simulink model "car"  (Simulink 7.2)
settings: Solver=ode15s  StartTime=0.0  StopTime=60  RelTol=1e-3
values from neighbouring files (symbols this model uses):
  A_a = 1.5    [modelparam.m]
  b_f = 0.1    [modelparam.m]
  b_t = 0.1    [modelparam.m]
  brake_gain = 1.0e3    (= 1000)    [modelparam.m]
  Bx = Kxk/(Cx*Dx)    (= 12.5)    [modelparam.m]
  c_c = 30    [modelparam.m]
  c_d = 1    [modelparam.m]
  c_p = 15    [modelparam.m]
  c_r = 0.015    [modelparam.m]
  c_w = 0.30    (= 0.3)    [modelparam.m]
  Cx = 1.2    [modelparam.m]
  Dx = muX*Fz    (= 5886)    [modelparam.m]
  Ex = 0.8    [modelparam.m]
  g = 9.81    [modelparam.m]
  gearInertia = [0.13 0.09 0.07 0.05 0.04]    [modelparam.m]
  gearNumber = [1 2 3 4 5]    [modelparam.m]
  gearRatio = [3.4 2.2 1.5 1.1 0.9]    [modelparam.m]
  i_f = 3.4    [modelparam.m]
  init_d = init_v/r_w/3.6    (= 27.7777777778)    [modelparam.m]
  init_e = init_t*gearRatio(2)    [modelparam.m]
  init_f = init_d    (= 27.7777777778)    [modelparam.m]
  init_t = init_f*i_f    (= 94.4444444444)    [modelparam.m]
  init_T = 0    [modelparam.m]
  J_e = 0.2    [modelparam.m]
  J_f = 0.1    [modelparam.m]
  J_w = 0.6    [modelparam.m]
  k_c = 10e3    (= 10000)    [modelparam.m]
  k_d = 1e3    (= 1000)    [modelparam.m]
  k_p = 0.5e4    (= 5000)    [modelparam.m]
  mass = 1.5e3    (= 1500)    [modelparam.m]
  N_max = 7e3*pi/30    (= 733.038285838)    [modelparam.m]
  position = [0 1e6]    [modelparam.m]
  r_w = 0.30    (= 0.3)    [modelparam.m]
  Rho_a = 1.29    [modelparam.m]
  slope = [0 0]    [modelparam.m]
  T_max = 400    [modelparam.m]
  tau_d = 1e-3    (= 0.001)    [modelparam.m]
  tau_e = 0.1    [modelparam.m]
libraries: simulink x4

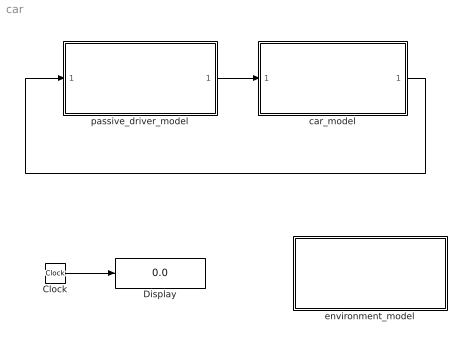
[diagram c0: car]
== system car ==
  Clock : Clock
  Display : Display
  car_model : Subsystem
  environment_model : Subsystem  AncestorBlock=capsim_lib/Environment/environment_model_jofr1  mask{Tamb=0, Pamb=0, pos=position, slope=slope}
      mask prompts: Tamb "Ambient Temperature [K]"; Pamb "Ambient Pressure [Pa]"; pos "positionvector in slope map [m]"; slope "slopevector in slope map [rad]"
      mask help: Environment settings
  passive_driver_model : Subsystem  AncestorBlock=capsim_lib/Driver/driver_model_template
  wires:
  car_model/1(vehicle fb out) -> passive_driver_model/1(vehicle fb in)
  passive_driver_model/1(driver cmd out) -> car_model/1(driver cmd in)
  Clock/1 -> Display/1

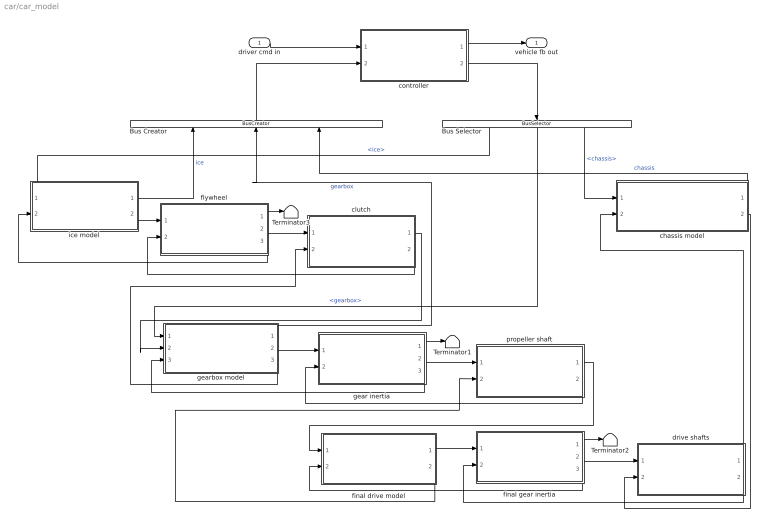
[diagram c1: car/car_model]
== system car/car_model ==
  driver cmd in : Inport  OutDataType=sfix(16)  OutScaling=2^0
  Bus Creator : BusCreator  Orientation=up  Inputs=3
  Bus Selector : BusSelector  Orientation=down  OutputSignals=ice,gearbox,chassis
  Terminator1 : Terminator
  Terminator2 : Terminator
  Terminator3 : Terminator
  chassis model : Subsystem  AncestorBlock=capsim_lib/Chassis/chassis_model_template
  clutch : Subsystem  AncestorBlock=capsim_lib/MechConverter/mechconverter_simple1_std  mask{mass=0, inertia=0, k_c=k_c, c_c=c_c}
      mask prompts: mass "Component mass [kg]"; inertia "Inertia [kg*m2]"; k_c "stiffness [Nm/rad]"; c_c "damping [Nms/rad]"
      mask help: Inertia
  controller : Subsystem  AncestorBlock=capsim_lib/Controller/controller_template
  drive shafts : Subsystem  AncestorBlock=capsim_lib/MechConverter/mechconverter_simple1_std  mask{mass=0, inertia=0, k_d=k_d, c_d=c_d}
      mask prompts: mass "Component mass [kg]"; inertia "Inertia [kg*m2]"; k_d "stiffness [Nm/rad]"; c_d "damping [Nms/rad]"
      mask help: Inertia
  final drive model : Subsystem  AncestorBlock=capsim_lib/Gearbox/gearbox_template
  final gear inertia : Subsystem  AncestorBlock=capsim_lib/Inertia/inertia_simple1_std  mask{mass=0, inertia=0, speedinit=init_f, angleinit=0}
      mask prompts: mass "Component mass [kg]"; inertia "Inertia [kg*m2]"; speedinit "Initial speed [rad/s]"; angleinit "Initial angle [rad]"
      mask help: Inertia
  flywheel : Subsystem  AncestorBlock=capsim_lib/Inertia/inertia_simple1_std  mask{mass=0, inertia=0, speedinit=init_e, angleinit=0}
      mask prompts: mass "Component mass [kg]"; inertia "Inertia [kg*m2]"; speedinit "Initial speed [rad/s]"; angleinit "Initial angle [rad]"
      mask help: Inertia
  gear inertia : Subsystem  AncestorBlock=capsim_lib/Inertia/inertia_simple1_std  mask{mass=0, inertia=0, speedinit=init_t, angleinit=0}
      mask prompts: mass "Component mass [kg]"; inertia "Inertia [kg*m2]"; speedinit "Initial speed [rad/s]"; angleinit "Initial angle [rad]"
      mask help: Inertia
  gearbox model : Subsystem  AncestorBlock=capsim_lib/Gearbox/gearbox_template
  ice model : Subsystem  AncestorBlock=capsim_lib/ICE/ice_model_template
  propeller shaft : Subsystem  AncestorBlock=capsim_lib/MechConverter/mechconverter_simple1_std  mask{mass=0, inertia=0, k_p=k_p, c_p=c_p}
      mask prompts: mass "Component mass [kg]"; inertia "Inertia [kg*m2]"; k_p "stiffness [Nm/rad]"; c_p "damping [Nms/rad]"
      mask help: Inertia
  vehicle fb out : Outport  OutDataType=sfix(16)  OutScaling=2^0
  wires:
  controller/1(vehicle fb out) -> vehicle fb out/1
  driver cmd in/1 -> controller/1(driver cmd in)
  controller/2(cmd out) -> Bus Selector/1
  Bus Creator/1 -> controller/2(sensor in)
  Bus Selector/1 -> ice model/1(cmd in)  "<ice>"
  Bus Selector/3 -> chassis model/1(cmd in)  "<chassis>"
  chassis model/1(sensor out) -> Bus Creator/3  "chassis"
  ice model/2(mech power out [Nm]) -> flywheel/1(mech in [Nm])
  flywheel/3(mech fb out [rad/s]) -> ice model/2(mech fb in [rad/s])
  flywheel/2(mech out [rad/s]) -> clutch/1(mech in [rad/s])
  clutch/2(mech fb out [Nm]) -> flywheel/2(mech fb in [Nm])
  clutch/1(mech out [Nm]) -> gearbox model/2(mech power in [Nm])
  gearbox model/2(mech power out [Nm]) -> gear inertia/1(mech in [Nm])
  gearbox model/3(mech fb out [rad/s]) -> clutch/2(mech fb in [rad/s])
  gear inertia/3(mech fb out [rad/s]) -> gearbox model/3(mech fb in [rad/s])
  gear inertia/2(mech out [rad/s]) -> propeller shaft/1(mech in [rad/s])
  propeller shaft/2(mech fb out [Nm]) -> gear inertia/2(mech fb in [Nm])
  propeller shaft/1(mech out [Nm]) -> final drive model/1(mech power in [Nm])
  final drive model/2(mech fb out [rad/s]) -> propeller shaft/2(mech fb in [rad/s])
  final drive model/1(mech power out [Nm]) -> final gear inertia/1(mech in [Nm])
  final gear inertia/2(mech out [rad/s]) -> drive shafts/1(mech in [rad/s])
  final gear inertia/3(mech fb out [rad/s]) -> final drive model/2(mech fb in [rad/s])
  drive shafts/1(mech out [Nm]) -> chassis model/2(mech power in [Nm])
  drive shafts/2(mech fb out [Nm]) -> final gear inertia/2(mech fb in [Nm])
  chassis model/2(mech fb out [rad/s]) -> drive shafts/2(mech fb in [rad/s])
  ice model/1(sensor out) -> Bus Creator/1  "ice"
  flywheel/1(sensor out) -> Terminator3/1
  gearbox model/1(sensor out) -> Bus Creator/2  "gearbox"
  gear inertia/1(sensor out) -> Terminator1/1
  final gear inertia/1(sensor out) -> Terminator2/1
  Bus Selector/2 -> gearbox model/1(cmd in)  "<gearbox>"

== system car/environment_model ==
  Compare To Constant : simulink/Logic and Bit Operations/Compare To Constant  SystemSampleTime=-1  relop=<  const=1  LogicOutDataTypeMode=uint8  ZeroCross=off
  Compare To Constant1 : simulink/Logic and Bit Operations/Compare To Constant  SystemSampleTime=-1  relop=<  const=1  LogicOutDataTypeMode=uint8  ZeroCross=off
  Constant2 : Constant  Value=pos(end)  OutDataType=sfix(16)  OutScaling=2^0
  Integrator : Integrator
  Logical Operator : Logic  Operator=OR  Inputs=3  AllPortsSameDT=off  OutDataTypeMode=boolean  OutDataTypeStr=boolean
  Relational Operator : RelationalOperator
  Stop Simulation1 : Stop
  To Workspace2 : ToWorkspace  VariableName=environmentout  SampleTime=-1  SaveFormat=Array
  slope as function of the distance : Lookup  InputValues=pos  Table=slope  LookUpMeth=Interpolation-Use End Values  OutDataType=sfix(16)  OutScaling=2^0
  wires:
  [speed] -> Integrator/1, Compare To Constant/1
  Integrator/1 -> slope as function of the distance/1, Relational Operator/1  "distance"
  slope as function of the distance/1 -> [slope], To Workspace2/1
  Constant2/1 -> Relational Operator/2
  Logical Operator/1 -> Stop Simulation1/1
  Relational Operator/1 -> Logical Operator/1
  Compare To Constant/1 -> Logical Operator/2
  [wheelspeed] -> Compare To Constant1/1
  Compare To Constant1/1 -> Logical Operator/3

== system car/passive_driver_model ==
  vehicle fb in : Inport  OutDataType=sfix(16)  OutScaling=2^0
  Bus Creator : BusCreator  Inputs=1
  Bus Selector : BusSelector  OutputSignals=velocity [m/s]
  From Workspace2 : FromWorkspace  VariableName=[InputT InputU]  SampleTime=0
  Terminator : Terminator
  driver cmd out : Outport  OutDataType=sfix(16)  OutScaling=2^0
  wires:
  vehicle fb in/1 -> Bus Selector/1
  Bus Creator/1 -> driver cmd out/1
  Bus Selector/1 -> Terminator/1  "<velocity [m/s]>"
  From Workspace2/1 -> Bus Creator/1  "Torque demand [%]"

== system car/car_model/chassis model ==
  cmd in : Inport  OutDataType=sfix(16)  OutScaling=2^0
  mech power in [Nm] : Inport  Port=2  OutDataType=sfix(16)  OutScaling=2^0
  chassis : Subsystem  mask{g=g, mass=mass, J_w=J_w, r_w=r_w, init_d=init_d, c_w=c_w, A_a=A_a, Rho_a=Rho_a, c_r=c_r, Bx=Bx, Cx=Cx, Dx=Dx, Ex=Ex}
      mask prompts: g "gravity constant [m/s^2]"; mass "vehicle mass [kg]"; J_w "wheel inertia [kg m^2]"; r_w "wheel radius [m]"; init_d "initial drive shaft speed [rad/s]"; c_w "air drag coefficient [-]"; A_a "max. vehicle cross section area [m^2]"; Rho_a "Air density [kg/m^3]"; c_r "rolling resistance coefficient [-]"; Bx "Magic Bx"; Cx "Magic Cx"; Dx "Magic Dx"; Ex "Magic Ex"
  local controller : Subsystem  mask{brake_gain=brake_gain}
      mask prompts: brake_gain "brake gain [Nm]"
  sensor out : Outport  OutDataType=sfix(16)  OutScaling=2^0
  mech fb out [rad/s] : Outport  Port=2  OutDataType=sfix(16)  OutScaling=2^0
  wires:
  local controller/2(ctrl out) -> chassis/1(ctrl in)
  cmd in/1 -> local controller/1(cmd in)
  local controller/1(sensor out) -> sensor out/1
  chassis/1(sensor out) -> local controller/2(sensor in)
  mech power in [Nm]/1 -> chassis/2(mech power in [Nm])
  chassis/2(mech fb out [rad/s]) -> mech fb out [rad/s]/1

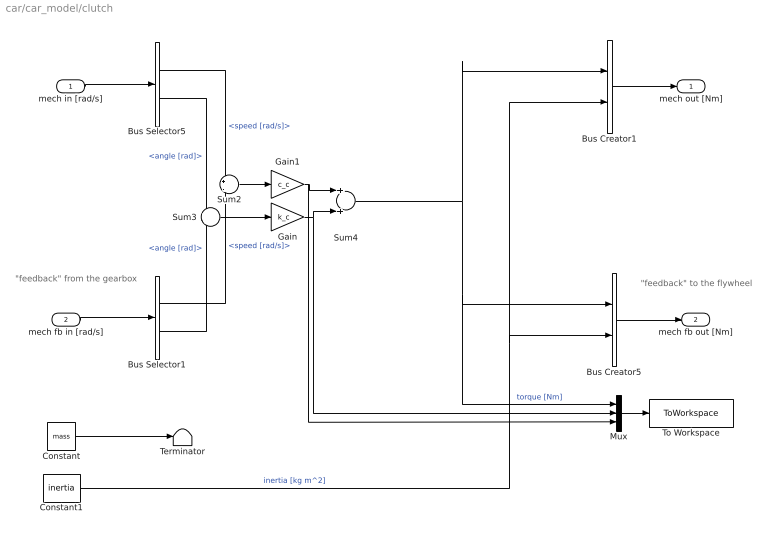
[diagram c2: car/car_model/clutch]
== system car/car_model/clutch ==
  note: "feedback" from the gearbox
  note: "feedback" to the flywheel
  mech in [rad/s] : Inport  OutDataType=sfix(16)  OutScaling=2^0
  mech fb in [rad/s] : Inport  Port=2  OutDataType=sfix(16)  OutScaling=2^0
  Bus Creator1 : BusCreator  Inputs=2
  Bus Creator5 : BusCreator  Inputs=2
  Bus Selector1 : BusSelector  OutputSignals=speed [rad/s],angle [rad]
  Bus Selector5 : BusSelector  OutputSignals=speed [rad/s],angle [rad]
  Constant : Constant  Value=mass  OutDataType=sfix(16)  OutScaling=2^0
  Constant1 : Constant  Value=inertia  OutDataType=sfix(16)  OutScaling=2^0
  Gain : Gain  Gain=k_c  ParameterDataType=sfix(16)  ParameterScaling=2^0  OutDataType=sfix(16)  OutScaling=2^0
  Gain1 : Gain  Gain=c_c  ParameterDataType=sfix(16)  ParameterScaling=2^0  OutDataType=sfix(16)  OutScaling=2^0
  Mux : Mux  Inputs=3
  Sum2 : Sum  Inputs=+|-  OutDataType=sfix(16)  OutScaling=2^0
  Sum3 : Sum  Inputs=+|-  OutDataType=sfix(16)  OutScaling=2^0
  Sum4 : Sum  OutDataType=sfix(16)  OutScaling=2^0
  Terminator : Terminator
  To Workspace : ToWorkspace  VariableName=clutchout  SampleTime=-1  SaveFormat=Array
  mech out [Nm] : Outport  OutDataType=sfix(16)  OutScaling=2^0
  mech fb out [Nm] : Outport  Port=2  OutDataType=sfix(16)  OutScaling=2^0
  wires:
  mech in [rad/s]/1 -> Bus Selector5/1
  mech fb in [rad/s]/1 -> Bus Selector1/1
  Mux/1 -> To Workspace/1
  Constant/1 -> Terminator/1
  Bus Creator5/1 -> mech fb out [Nm]/1
  Bus Creator1/1 -> mech out [Nm]/1
  Bus Selector5/1 -> Sum2/1  "<speed [rad/s]>"
  Bus Selector5/2 -> Sum3/1  "<angle [rad]>"
  Bus Selector1/1 -> Sum2/2  "<speed [rad/s]>"
  Bus Selector1/2 -> Sum3/2  "<angle [rad]>"
  Sum2/1 -> Gain1/1
  Sum3/1 -> Gain/1
  Gain1/1 -> Sum4/1, Mux/3
  Gain/1 -> Sum4/2, Mux/2
  Sum4/1 -> Bus Creator1/1, Bus Creator5/1, Mux/1  "torque [Nm]"
  Constant1/1 -> Bus Creator5/2, Bus Creator1/2  "inertia [kg m^2]"

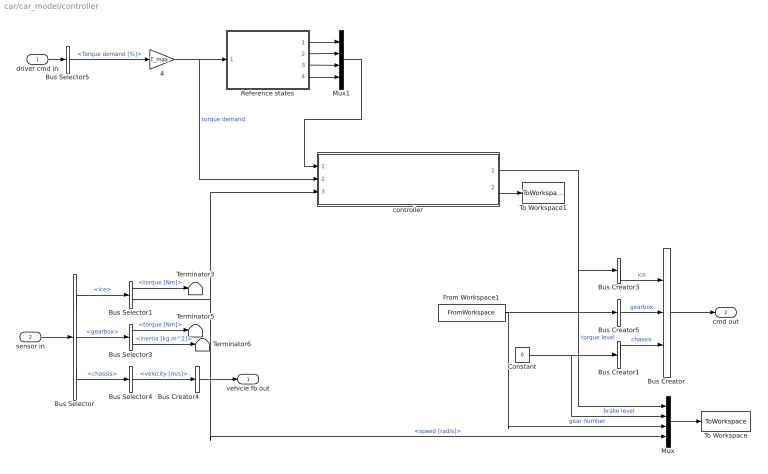
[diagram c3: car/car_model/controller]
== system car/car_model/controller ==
  driver cmd in : Inport  OutDataType=sfix(16)  OutScaling=2^0
  sensor in : Inport  Port=2  OutDataType=sfix(16)  OutScaling=2^0
  4 : Gain  Gain=T_max  ParameterDataType=sfix(16)  ParameterScaling=2^0  OutDataType=sfix(16)  OutScaling=2^0
  Bus Creator : BusCreator  Inputs=3
  Bus Creator{1,3..5} (4 alike) : BusCreator  Inputs=1
  Bus Selector : BusSelector  OutputSignals=ice,gearbox,chassis
  Bus Selector1 : BusSelector  OutputSignals=torque [Nm],speed [rad/s]
  Bus Selector3 : BusSelector  OutputSignals=torque [Nm],inertia [kg m^2]
  Bus Selector4 : BusSelector  OutputSignals=velocity [m/s]
  Bus Selector5 : BusSelector  OutputSignals=Torque demand [%]
  Constant : Constant  Value=0  OutDataType=sfix(16)  OutScaling=2^0
  From Workspace1 : FromWorkspace  VariableName=[InputT InputG]  SampleTime=0
  Mux : Mux
  Mux1 : Mux
  Reference states : Subsystem
  Terminator3 : Terminator
  Terminator5 : Terminator
  Terminator6 : Terminator
  To Workspace : ToWorkspace  VariableName=controllerout  SampleTime=-1  SaveFormat=Array
  To Workspace1 : ToWorkspace  VariableName=obsstates  SampleTime=-1  SaveFormat=Array
  controller : Subsystem
  vehicle fb out : Outport  OutDataType=sfix(16)  OutScaling=2^0
  cmd out : Outport  Port=2  OutDataType=sfix(16)  OutScaling=2^0
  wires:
  Bus Creator/1 -> cmd out/1
  Bus Creator3/1 -> Bus Creator/1  "ice"
  sensor in/1 -> Bus Selector/1
  Bus Selector/1 -> Bus Selector1/1  "<ice>"
  driver cmd in/1 -> Bus Selector5/1
  Bus Creator4/1 -> vehicle fb out/1
  Bus Selector5/1 -> 4/1  "<Torque demand [%]>"
  Bus Selector3/1 -> Terminator5/1  "<torque [Nm]>"
  Bus Selector3/2 -> Terminator6/1  "<inertia [kg m^2]>"
  Mux/1 -> To Workspace/1
  Bus Creator1/1 -> Bus Creator/3  "chassis"
  Bus Selector/2 -> Bus Selector3/1  "<gearbox>"
  Bus Selector/3 -> Bus Selector4/1  "<chassis>"
  Bus Selector1/1 -> Terminator3/1  "<torque [Nm]>"
  Bus Selector1/2 -> Mux/4, controller/3(Engine speed sensor)  "<speed [rad/s]>"
  Bus Selector4/1 -> Bus Creator4/1  "<velocity [m/s]>"
  Constant/1 -> Bus Creator1/1, Mux/2  "brake level"
  From Workspace1/1 -> Bus Creator5/1, Mux/3  "gear number"
  Bus Creator5/1 -> Bus Creator/2  "gearbox"
  4/1 -> Reference states/1(In1), controller/2(Torque demand from driver)  "torque demand"
  Reference states/1(Drive shaft torsion [rad]) -> Mux1/1
  Reference states/2(Engine speed [rad/s]) -> Mux1/2
  Reference states/3(Wheel speed [rad/s]) -> Mux1/3
  Reference states/4(Engine torque [Nm]) -> Mux1/4
  Mux1/1 -> controller/1(x_ref)
  controller/1(Torque demand from controller) -> Mux/1, Bus Creator3/1  "torque level"
  controller/2(Observed states) -> To Workspace1/1

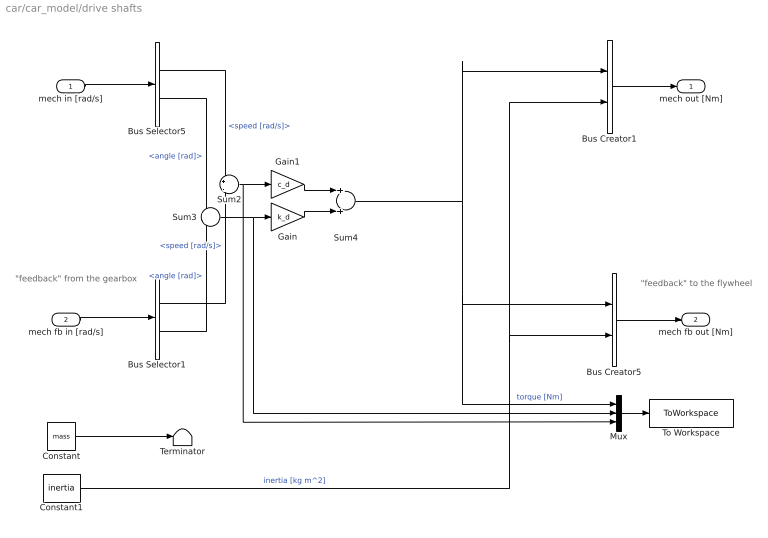
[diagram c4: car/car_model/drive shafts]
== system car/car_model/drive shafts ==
  note: "feedback" from the gearbox
  note: "feedback" to the flywheel
  mech in [rad/s] : Inport  OutDataType=sfix(16)  OutScaling=2^0
  mech fb in [rad/s] : Inport  Port=2  OutDataType=sfix(16)  OutScaling=2^0
  Bus Creator1 : BusCreator  Inputs=2
  Bus Creator5 : BusCreator  Inputs=2
  Bus Selector1 : BusSelector  OutputSignals=speed [rad/s],angle [rad]
  Bus Selector5 : BusSelector  OutputSignals=speed [rad/s],angle [rad]
  Constant : Constant  Value=mass  OutDataType=sfix(16)  OutScaling=2^0
  Constant1 : Constant  Value=inertia  OutDataType=sfix(16)  OutScaling=2^0
  Gain : Gain  Gain=k_d  ParameterDataType=sfix(16)  ParameterScaling=2^0  OutDataType=sfix(16)  OutScaling=2^0
  Gain1 : Gain  Gain=c_d  ParameterDataType=sfix(16)  ParameterScaling=2^0  OutDataType=sfix(16)  OutScaling=2^0
  Mux : Mux  Inputs=3
  Sum2 : Sum  Inputs=+|-  OutDataType=sfix(16)  OutScaling=2^0
  Sum3 : Sum  Inputs=+|-  OutDataType=sfix(16)  OutScaling=2^0
  Sum4 : Sum  OutDataType=sfix(16)  OutScaling=2^0
  Terminator : Terminator
  To Workspace : ToWorkspace  VariableName=driveshaftsout  SampleTime=-1  SaveFormat=Array
  mech out [Nm] : Outport  OutDataType=sfix(16)  OutScaling=2^0
  mech fb out [Nm] : Outport  Port=2  OutDataType=sfix(16)  OutScaling=2^0
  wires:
  mech in [rad/s]/1 -> Bus Selector5/1
  mech fb in [rad/s]/1 -> Bus Selector1/1
  Mux/1 -> To Workspace/1
  Constant/1 -> Terminator/1
  Bus Creator5/1 -> mech fb out [Nm]/1
  Bus Creator1/1 -> mech out [Nm]/1
  Bus Selector5/1 -> Sum2/1  "<speed [rad/s]>"
  Bus Selector5/2 -> Sum3/1  "<angle [rad]>"
  Bus Selector1/1 -> Sum2/2  "<speed [rad/s]>"
  Bus Selector1/2 -> Sum3/2  "<angle [rad]>"
  Sum2/1 -> Gain1/1, Mux/3
  Sum3/1 -> Gain/1, Mux/2
  Gain1/1 -> Sum4/1
  Gain/1 -> Sum4/2
  Sum4/1 -> Bus Creator1/1, Bus Creator5/1, Mux/1  "torque [Nm]"
  Constant1/1 -> Bus Creator5/2, Bus Creator1/2  "inertia [kg m^2]"

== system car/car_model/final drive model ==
  mech power in [Nm] : Inport  OutDataType=sfix(16)  OutScaling=2^0
  mech fb in [rad/s] : Inport  Port=2  OutDataType=sfix(16)  OutScaling=2^0
  final_drive : Subsystem  mask{mass=0, inertia=J_f, b_f=b_f, i_f=i_f}
      mask prompts: mass "mass [kg]"; inertia "inertia [kg m^2]"; b_f "Damping [Nm s/rad]"; i_f "Ratio [-]"
  mech power out [Nm] : Outport  OutDataType=sfix(16)  OutScaling=2^0
  mech fb out [rad/s] : Outport  Port=2  OutDataType=sfix(16)  OutScaling=2^0
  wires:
  mech fb in [rad/s]/1 -> final_drive/2(mech fb in [rad/s])
  final_drive/1(mech power out [Nm]) -> mech power out [Nm]/1
  mech power in [Nm]/1 -> final_drive/1(mech power in [Nm])
  final_drive/2(mech fb out [rad/s]) -> mech fb out [rad/s]/1

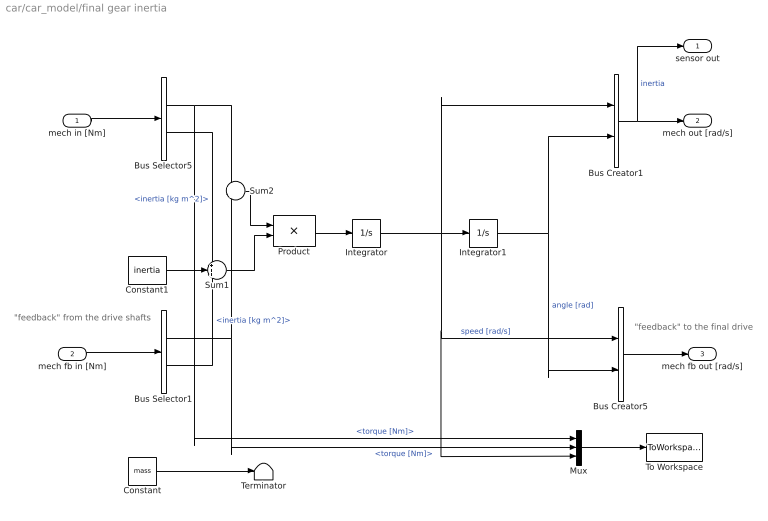
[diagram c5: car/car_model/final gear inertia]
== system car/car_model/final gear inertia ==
  note: "feedback" to the final drive
  note: "feedback" from the drive shafts
  mech in [Nm] : Inport  OutDataType=sfix(16)  OutScaling=2^0
  mech fb in [Nm] : Inport  Port=2  OutDataType=sfix(16)  OutScaling=2^0
  Bus Creator1 : BusCreator  Inputs=2
  Bus Creator5 : BusCreator  Inputs=2
  Bus Selector1 : BusSelector  OutputSignals=torque [Nm],inertia [kg m^2]
  Bus Selector5 : BusSelector  OutputSignals=torque [Nm],inertia [kg m^2]
  Constant : Constant  Value=mass  OutDataType=sfix(16)  OutScaling=2^0
  Constant1 : Constant  Value=inertia  OutDataType=sfix(16)  OutScaling=2^0
  Integrator : Integrator  InitialCondition=speedinit
  Integrator1 : Integrator  InitialCondition=angleinit
  Mux : Mux  Inputs=3
  Product : Product  Inputs=*/  OutDataType=sfix(16)  OutScaling=2^0
  Sum1 : Sum  Inputs=+++  OutDataType=sfix(16)  OutScaling=2^0
  Sum2 : Sum  Inputs=+|-  OutDataType=sfix(16)  OutScaling=2^0
  Terminator : Terminator
  To Workspace : ToWorkspace  VariableName=finalgearout  SampleTime=-1  SaveFormat=Array
  sensor out : Outport  OutDataType=sfix(16)  OutScaling=2^0
  mech out [rad/s] : Outport  Port=2  OutDataType=sfix(16)  OutScaling=2^0
  mech fb out [rad/s] : Outport  Port=3  OutDataType=sfix(16)  OutScaling=2^0
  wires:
  Constant1/1 -> Sum1/2
  Bus Selector1/2 -> Sum1/3  "<inertia [kg m^2]>"
  Bus Selector1/1 -> Sum2/2, Mux/2  "<torque [Nm]>"
  Bus Selector5/2 -> Sum1/1  "<inertia [kg m^2]>"
  Bus Selector5/1 -> Sum2/1, Mux/1  "<torque [Nm]>"
  Bus Creator1/1 -> sensor out/1, mech out [rad/s]/1  "inertia"
  Bus Creator5/1 -> mech fb out [rad/s]/1
  mech fb in [Nm]/1 -> Bus Selector1/1
  Constant/1 -> Terminator/1
  mech in [Nm]/1 -> Bus Selector5/1
  Integrator1/1 -> Bus Creator5/2, Bus Creator1/2  "angle [rad]"
  Integrator/1 -> Bus Creator1/1, Integrator1/1, Bus Creator5/1, Mux/3  "speed [rad/s]"
  Product/1 -> Integrator/1
  Sum1/1 -> Product/2
  Sum2/1 -> Product/1
  Mux/1 -> To Workspace/1

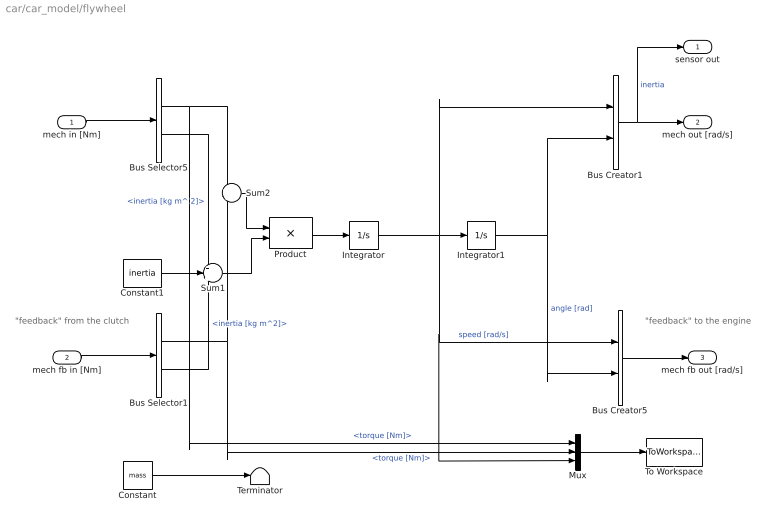
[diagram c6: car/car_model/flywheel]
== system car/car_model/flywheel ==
  note: "feedback" to the engine
  note: "feedback" from the clutch
  mech in [Nm] : Inport  OutDataType=sfix(16)  OutScaling=2^0
  mech fb in [Nm] : Inport  Port=2  OutDataType=sfix(16)  OutScaling=2^0
  Bus Creator1 : BusCreator  Inputs=2
  Bus Creator5 : BusCreator  Inputs=2
  Bus Selector1 : BusSelector  OutputSignals=torque [Nm],inertia [kg m^2]
  Bus Selector5 : BusSelector  OutputSignals=torque [Nm],inertia [kg m^ 2]
  Constant : Constant  Value=mass  OutDataType=sfix(16)  OutScaling=2^0
  Constant1 : Constant  Value=inertia  OutDataType=sfix(16)  OutScaling=2^0
  Integrator : Integrator  InitialCondition=speedinit
  Integrator1 : Integrator  InitialCondition=angleinit
  Mux : Mux  Inputs=3
  Product : Product  Inputs=*/  OutDataType=sfix(16)  OutScaling=2^0
  Sum1 : Sum  Inputs=+++  OutDataType=sfix(16)  OutScaling=2^0
  Sum2 : Sum  Inputs=+|-  OutDataType=sfix(16)  OutScaling=2^0
  Terminator : Terminator
  To Workspace : ToWorkspace  VariableName=flywheelout  SampleTime=-1  SaveFormat=Array
  sensor out : Outport  OutDataType=sfix(16)  OutScaling=2^0
  mech out [rad/s] : Outport  Port=2  OutDataType=sfix(16)  OutScaling=2^0
  mech fb out [rad/s] : Outport  Port=3  OutDataType=sfix(16)  OutScaling=2^0
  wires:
  Mux/1 -> To Workspace/1
  Sum2/1 -> Product/1
  Sum1/1 -> Product/2
  Product/1 -> Integrator/1
  Integrator/1 -> Mux/3, Bus Creator5/1, Integrator1/1, Bus Creator1/1  "speed [rad/s]"
  Integrator1/1 -> Bus Creator5/2, Bus Creator1/2  "angle [rad]"
  mech in [Nm]/1 -> Bus Selector5/1
  Constant/1 -> Terminator/1
  mech fb in [Nm]/1 -> Bus Selector1/1
  Bus Creator5/1 -> mech fb out [rad/s]/1
  Bus Creator1/1 -> mech out [rad/s]/1, sensor out/1  "inertia"
  Bus Selector5/1 -> Mux/1, Sum2/1  "<torque [Nm]>"
  Bus Selector5/2 -> Sum1/1  "<inertia [kg m^ 2]>"
  Bus Selector1/1 -> Mux/2, Sum2/2  "<torque [Nm]>"
  Bus Selector1/2 -> Sum1/3  "<inertia [kg m^2]>"
  Constant1/1 -> Sum1/2

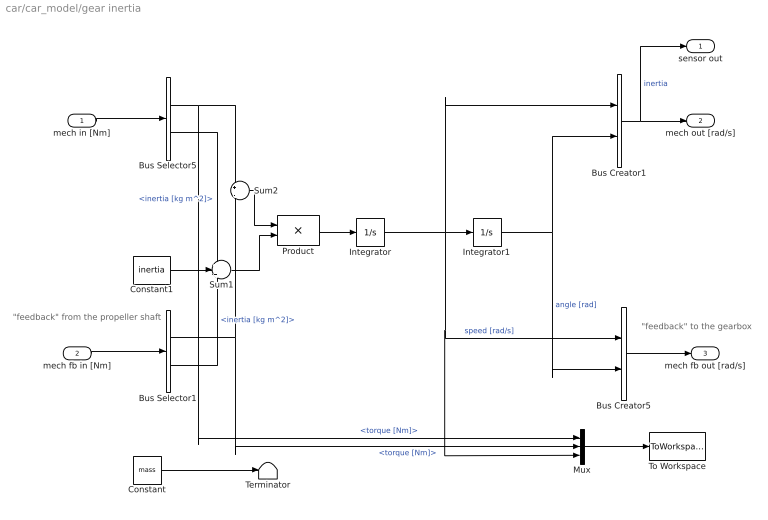
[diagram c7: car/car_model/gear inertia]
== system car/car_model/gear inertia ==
  note: "feedback" from the propeller shaft
  note: "feedback" to the gearbox
  mech in [Nm] : Inport  OutDataType=sfix(16)  OutScaling=2^0
  mech fb in [Nm] : Inport  Port=2  OutDataType=sfix(16)  OutScaling=2^0
  Bus Creator1 : BusCreator  Inputs=2
  Bus Creator5 : BusCreator  Inputs=2
  Bus Selector1 : BusSelector  OutputSignals=torque [Nm],inertia [kg m^2]
  Bus Selector5 : BusSelector  OutputSignals=torque [Nm],inertia [kg m^2]
  Constant : Constant  Value=mass  OutDataType=sfix(16)  OutScaling=2^0
  Constant1 : Constant  Value=inertia  OutDataType=sfix(16)  OutScaling=2^0
  Integrator : Integrator  InitialCondition=speedinit
  Integrator1 : Integrator  InitialCondition=angleinit
  Mux : Mux  Inputs=3
  Product : Product  Inputs=*/  OutDataType=sfix(16)  OutScaling=2^0
  Sum1 : Sum  Inputs=+++  OutDataType=sfix(16)  OutScaling=2^0
  Sum2 : Sum  Inputs=+|-  OutDataType=sfix(16)  OutScaling=2^0
  Terminator : Terminator
  To Workspace : ToWorkspace  VariableName=gearinertiaout  SampleTime=-1  SaveFormat=Array
  sensor out : Outport  OutDataType=sfix(16)  OutScaling=2^0
  mech out [rad/s] : Outport  Port=2  OutDataType=sfix(16)  OutScaling=2^0
  mech fb out [rad/s] : Outport  Port=3  OutDataType=sfix(16)  OutScaling=2^0
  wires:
  Mux/1 -> To Workspace/1
  Sum2/1 -> Product/1
  Sum1/1 -> Product/2
  Product/1 -> Integrator/1
  Integrator/1 -> Mux/3, Bus Creator5/1, Integrator1/1, Bus Creator1/1  "speed [rad/s]"
  Integrator1/1 -> Bus Creator5/2, Bus Creator1/2  "angle [rad]"
  mech in [Nm]/1 -> Bus Selector5/1
  Constant/1 -> Terminator/1
  mech fb in [Nm]/1 -> Bus Selector1/1
  Bus Creator5/1 -> mech fb out [rad/s]/1
  Bus Creator1/1 -> mech out [rad/s]/1, sensor out/1  "inertia"
  Bus Selector5/1 -> Mux/1, Sum2/1  "<torque [Nm]>"
  Bus Selector5/2 -> Sum1/1  "<inertia [kg m^2]>"
  Bus Selector1/1 -> Mux/2, Sum2/2  "<torque [Nm]>"
  Bus Selector1/2 -> Sum1/3  "<inertia [kg m^2]>"
  Constant1/1 -> Sum1/2

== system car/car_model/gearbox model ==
  cmd in : Inport  OutDataType=sfix(16)  OutScaling=2^0
  mech power in [Nm] : Inport  Port=2  OutDataType=sfix(16)  OutScaling=2^0
  mech fb in [rad/s] : Inport  Port=3  OutDataType=sfix(16)  OutScaling=2^0
  gearbox : Subsystem  mask{mass=0, inertia=0, b_t=b_t}
      mask prompts: mass "mass [kg]"; inertia "inertia [kg m^2]"; b_t "Damping [Nm s/rad]"
  local controller : Subsystem  mask{gearNumber=gearNumber, gearRatio=gearRatio, gearInertia=gearInertia}
      mask prompts: gearNumber "gear number vector"; gearRatio "gear ratio vector"; gearInertia "gear inertia vector"
  sensor out : Outport  OutDataType=sfix(16)  OutScaling=2^0
  mech power out [Nm] : Outport  Port=2  OutDataType=sfix(16)  OutScaling=2^0
  mech fb out [rad/s] : Outport  Port=3  OutDataType=sfix(16)  OutScaling=2^0
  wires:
  gearbox/3(mech fb out [rad/s]) -> mech fb out [rad/s]/1
  mech power in [Nm]/1 -> gearbox/2(mech power in [Nm])
  gearbox/2(mech power out [Nm]) -> mech power out [Nm]/1
  mech fb in [rad/s]/1 -> gearbox/3(mech fb in [rad/s])
  gearbox/1(sensor out) -> local controller/2(sensor in)
  local controller/1(sensor out) -> sensor out/1
  cmd in/1 -> local controller/1(cmd in)
  local controller/2(ctrl) -> gearbox/1(ctrl)

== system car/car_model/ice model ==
  cmd in : Inport  OutDataType=sfix(16)  OutScaling=2^0
  mech fb in [rad/s] : Inport  Port=2  OutDataType=sfix(16)  OutScaling=2^0
  ice : Subsystem  mask{mass=0, inertia=J_e, tau_d=tau_d, tau_e=tau_e, init_T=init_T}
      mask prompts: mass "mass [kg]"; inertia "inertia [kg m^2]"; tau_d "time delay [s]"; tau_e "time constant [s]"; init_T "initial torque [Nm]"
  local controller : Subsystem  mask{T_max=T_max, N_max=N_max}
      mask prompts: T_max "maximum torque [Nm]"; N_max "maximum speed [rad/s]"
  sensor out : Outport  OutDataType=sfix(16)  OutScaling=2^0
  mech power out [Nm] : Outport  Port=2  OutDataType=sfix(16)  OutScaling=2^0
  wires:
  ice/2(mech power out [Nm]) -> mech power out [Nm]/1
  mech fb in [rad/s]/1 -> ice/2(mech fb in [rad/s])
  ice/1(sensor out) -> local controller/2(sensor in)
  local controller/1(sensor out) -> sensor out/1
  cmd in/1 -> local controller/1(cmd in)
  local controller/2(ctrl) -> ice/1(ctrl)

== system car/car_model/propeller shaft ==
  note: "feedback" to the flywheel
  note: "feedback" from the gearbox
  mech in [rad/s] : Inport  OutDataType=sfix(16)  OutScaling=2^0
  mech fb in [rad/s] : Inport  Port=2  OutDataType=sfix(16)  OutScaling=2^0
  Bus Creator1 : BusCreator  Inputs=2
  Bus Creator5 : BusCreator  Inputs=2
  Bus Selector1 : BusSelector  OutputSignals=speed [rad/s],angle [rad]
  Bus Selector5 : BusSelector  OutputSignals=speed [rad/s],angle [rad]
  Constant : Constant  Value=mass  OutDataType=sfix(16)  OutScaling=2^0
  Constant1 : Constant  Value=inertia  OutDataType=sfix(16)  OutScaling=2^0
  Gain : Gain  Gain=k_p  ParameterDataType=sfix(16)  ParameterScaling=2^0  OutDataType=sfix(16)  OutScaling=2^0
  Gain1 : Gain  Gain=c_p  ParameterDataType=sfix(16)  ParameterScaling=2^0  OutDataType=sfix(16)  OutScaling=2^0
  Mux : Mux  Inputs=3
  Sum2 : Sum  Inputs=+|-  OutDataType=sfix(16)  OutScaling=2^0
  Sum3 : Sum  Inputs=+|-  OutDataType=sfix(16)  OutScaling=2^0
  Sum4 : Sum  OutDataType=sfix(16)  OutScaling=2^0
  Terminator : Terminator
  To Workspace : ToWorkspace  VariableName=propellershaftout  SampleTime=-1  SaveFormat=Array
  mech out [Nm] : Outport  OutDataType=sfix(16)  OutScaling=2^0
  mech fb out [Nm] : Outport  Port=2  OutDataType=sfix(16)  OutScaling=2^0
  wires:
  Constant1/1 -> Bus Creator1/2, Bus Creator5/2  "inertia [kg m^2]"
  Sum4/1 -> Mux/1, Bus Creator5/1, Bus Creator1/1  "torque [Nm]"
  Gain/1 -> Sum4/2, Mux/2
  Gain1/1 -> Sum4/1, Mux/3
  Sum3/1 -> Gain/1
  Sum2/1 -> Gain1/1
  Bus Selector1/2 -> Sum3/2  "<angle [rad]>"
  Bus Selector1/1 -> Sum2/2  "<speed [rad/s]>"
  Bus Selector5/2 -> Sum3/1  "<angle [rad]>"
  Bus Selector5/1 -> Sum2/1  "<speed [rad/s]>"
  Bus Creator1/1 -> mech out [Nm]/1
  Bus Creator5/1 -> mech fb out [Nm]/1
  Constant/1 -> Terminator/1
  Mux/1 -> To Workspace/1
  mech fb in [rad/s]/1 -> Bus Selector1/1
  mech in [rad/s]/1 -> Bus Selector5/1

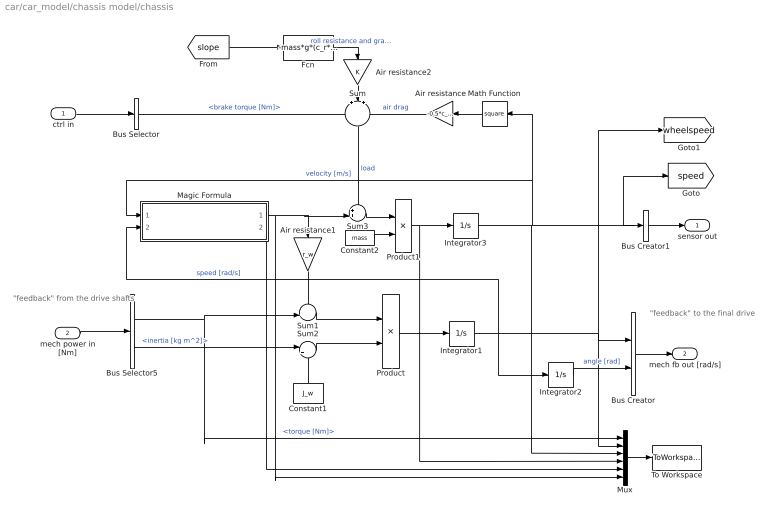
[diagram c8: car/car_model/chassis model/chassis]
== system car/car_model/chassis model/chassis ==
  note: "feedback" from the drive shafts
  note: "feedback" to the final drive
  ctrl in : Inport  OutDataType=sfix(16)  OutScaling=2^0
  mech power in [Nm] : Inport  Port=2  OutDataType=sfix(16)  OutScaling=2^0
  Air resistance : Gain  Orientation=left  Gain=-0.5*c_w*A_a*Rho_a  ParameterDataType=sfix(16)  ParameterScaling=2^0  OutDataType=sfix(16)  OutScaling=2^0
  Air resistance1 : Gain  Orientation=down  Gain=r_w  ParameterDataType=sfix(16)  ParameterScaling=2^0  OutDataType=sfix(16)  OutScaling=2^0
  Air resistance2 : Gain  Orientation=down  ParameterDataType=sfix(16)  ParameterScaling=2^0  OutDataType=sfix(16)  OutScaling=2^0
  Bus Creator : BusCreator  Inputs=2
  Bus Creator1 : BusCreator  Inputs=1
  Bus Selector : BusSelector  OutputSignals=brake torque [Nm]
  Bus Selector5 : BusSelector  OutputSignals=torque [Nm],inertia [kg m^2]
  Constant1 : Constant  Orientation=up  Value=J_w  OutDataType=sfix(16)  OutScaling=2^0
  Constant2 : Constant  Value=mass  OutDataType=sfix(16)  OutScaling=2^0
  Fcn : Fcn  Expr=-mass*g*(c_r*cos(u) + sin(u))
  Integrator1 : Integrator  InitialCondition=init_d
  Integrator2 : Integrator
  Integrator3 : Integrator  InitialCondition=init_d*r_w
  Magic Formula : Subsystem
  Math Function : Math  Orientation=left  Operator=square  OutDataType=sfix(16)  OutScaling=2^0
  Mux : Mux  Inputs=6
  Product : Product  Inputs=*/  OutDataType=sfix(16)  OutScaling=2^0
  Product1 : Product  Inputs=*/  OutDataType=sfix(16)  OutScaling=2^0
  Sum : Sum  Orientation=down  Inputs=+|+|+  OutDataType=sfix(16)  OutScaling=2^0
  Sum1 : Sum  Inputs=-+|  OutDataType=sfix(16)  OutScaling=2^0
  Sum2 : Sum  Inputs=|++  OutDataType=sfix(16)  OutScaling=2^0
  Sum3 : Sum  Inputs=++|  OutDataType=sfix(16)  OutScaling=2^0
  To Workspace : ToWorkspace  VariableName=chassisout  SampleTime=-1  SaveFormat=Array
  sensor out : Outport  OutDataType=sfix(16)  OutScaling=2^0
  mech fb out [rad/s] : Outport  Port=2  OutDataType=sfix(16)  OutScaling=2^0
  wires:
  Mux/1 -> To Workspace/1
  Integrator2/1 -> Bus Creator/2  "angle [rad]"
  Bus Selector5/2 -> Sum2/1  "<inertia [kg m^2]>"
  Bus Selector5/1 -> Mux/1, Sum1/2  "<torque [Nm]>"
  mech power in [Nm]/1 -> Bus Selector5/1
  Bus Creator/1 -> mech fb out [rad/s]/1
  ctrl in/1 -> Bus Selector/1
  [slope] -> Fcn/1
  Math Function/1 -> Air resistance/1
  Integrator1/1 -> Integrator2/1, Magic Formula/2(wheel speed [rad/s]), Mux/2, Bus Creator/1, [wheelspeed]  "speed [rad/s]"
  Air resistance/1 -> Sum/3  "air drag"
  Fcn/1 -> Air resistance2/1  "roll resistance and gravity"
  Bus Selector/1 -> Sum/1  "<brake torque [Nm]>"
  Bus Creator1/1 -> sensor out/1
  Sum2/1 -> Product/2
  Sum1/1 -> Product/1
  Product/1 -> Integrator1/1
  Constant1/1 -> Sum2/2
  Sum/1 -> Sum3/1  "load"
  Magic Formula/1(F_w [N]) -> Sum3/2, Air resistance1/1, Mux/6
  Sum3/1 -> Product1/1
  Constant2/1 -> Product1/2
  Product1/1 -> Integrator3/1, Mux/4
  Integrator3/1 -> Mux/3, Math Function/1, Magic Formula/1(forward velocity [m/s]), Bus Creator1/1, [speed]  "velocity [m/s]"
  Air resistance1/1 -> Sum1/1
  Magic Formula/2(slip ratio) -> Mux/5
  Air resistance2/1 -> Sum/2

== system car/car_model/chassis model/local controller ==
  cmd in : Inport  OutDataType=sfix(16)  OutScaling=2^0
  sensor in : Inport  Port=2  OutDataType=sfix(16)  OutScaling=2^0
  Bus Creator : BusCreator  Inputs=1
  Bus Selector : BusSelector  OutputSignals=brake level
  Saturation : Saturate  UpperLimit=1  LowerLimit=0
  brake_gain : Gain  Gain=-brake_gain  ParameterDataType=sfix(16)  ParameterScaling=2^0  OutDataType=sfix(16)  OutScaling=2^0
  sensor out : Outport  OutDataType=sfix(16)  OutScaling=2^0
  ctrl out : Outport  Port=2  OutDataType=sfix(16)  OutScaling=2^0
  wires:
  cmd in/1 -> Bus Selector/1
  Bus Selector/1 -> Saturation/1  "<brake level>"
  Saturation/1 -> brake_gain/1
  brake_gain/1 -> Bus Creator/1  "brake torque [Nm]"
  Bus Creator/1 -> ctrl out/1
  sensor in/1 -> sensor out/1

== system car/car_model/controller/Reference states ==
  In1 : Inport  OutDataType=sfix(16)  OutScaling=2^0
  1 : Gain  Gain=i_f*gearRatio(1)  ParameterDataType=sfix(16)  ParameterScaling=2^0  OutDataType=sfix(16)  OutScaling=2^0
  2 : Gain  Gain=1/tau_e  ParameterDataType=sfix(16)  ParameterScaling=2^0  OutDataType=sfix(16)  OutScaling=2^0
  5 : Gain  Gain=1/r_w  ParameterDataType=sfix(16)  ParameterScaling=2^0  OutDataType=sfix(16)  OutScaling=2^0
  6 : Gain  Gain=i_f*gearRatio(1)/k_d  ParameterDataType=sfix(16)  ParameterScaling=2^0  OutDataType=sfix(16)  OutScaling=2^0
  Add : Sum  Inputs=+-  OutDataType=sfix(16)  OutScaling=2^-10
  Fcn : Fcn  Expr=(i_f*gearRatio(1)/r_w*u(1)-0.5*Rho_a*c_w*A_a*u(2)^2-mass*g*c_r)/(mass+i_f^2*gearRatio(1)^2/r_w^2*J_e)
  Integrator : Integrator  InitialCondition=28/3.6
  Integrator1 : Integrator  InitialCondition=-8
  Mux6 : Mux  Inputs=2
  Drive shaft torsion [rad] : Outport  OutDataType=sfix(16)  OutScaling=2^0
  Engine speed [rad/s] : Outport  Port=2  OutDataType=sfix(16)  OutScaling=2^0
  Wheel speed [rad/s] : Outport  Port=3  OutDataType=sfix(16)  OutScaling=2^0
  Engine torque [Nm] : Outport  Port=4  OutDataType=sfix(16)  OutScaling=2^0
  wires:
  Fcn/1 -> Integrator/1
  Integrator/1 -> Mux6/2, 5/1  "v"
  Mux6/1 -> Fcn/1
  5/1 -> Wheel speed [rad/s]/1, 1/1
  6/1 -> Drive shaft torsion [rad]/1
  1/1 -> Engine speed [rad/s]/1
  Integrator1/1 -> Mux6/1, Engine torque [Nm]/1, 6/1, Add/2
  In1/1 -> Add/1
  Add/1 -> 2/1
  2/1 -> Integrator1/1

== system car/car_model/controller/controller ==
  note: Construct an observer for the vehicle using the engine speed sensor. Then use the given reference states (x_ref) and design a state feedback controller to damp the driveline oscillations.
  note: Connect your observed states hear to plot them in Figure 3
  x_ref : Inport  OutDataType=sfix(16)  OutScaling=2^0
  Torque demand from driver : Inport  Port=2  OutDataType=sfix(16)  OutScaling=2^0
  Engine speed sensor : Inport  Port=3  OutDataType=sfix(16)  OutScaling=2^0
  Ground : Ground
  Ground1 : Ground
  Manual Switch : simulink/Signal Routing/Manual Switch  SystemSampleTime=-1  sw=1  action=0  varsize=off
  Mux : Mux
  Terminator1 : Terminator
  Terminator3 : Terminator
  Torque demand from controller : Outport  OutDataType=sfix(16)  OutScaling=2^0
  Observed states : Outport  Port=2  OutDataType=sfix(16)  OutScaling=2^0
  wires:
  Torque demand from driver/1 -> Manual Switch/1
  Manual Switch/1 -> Torque demand from controller/1
  Engine speed sensor/1 -> Terminator3/1
  x_ref/1 -> Terminator1/1
  Ground/1 -> Manual Switch/2
  Ground1/1 -> Mux/1, Mux/2, Mux/3, Mux/4
  Mux/1 -> Observed states/1

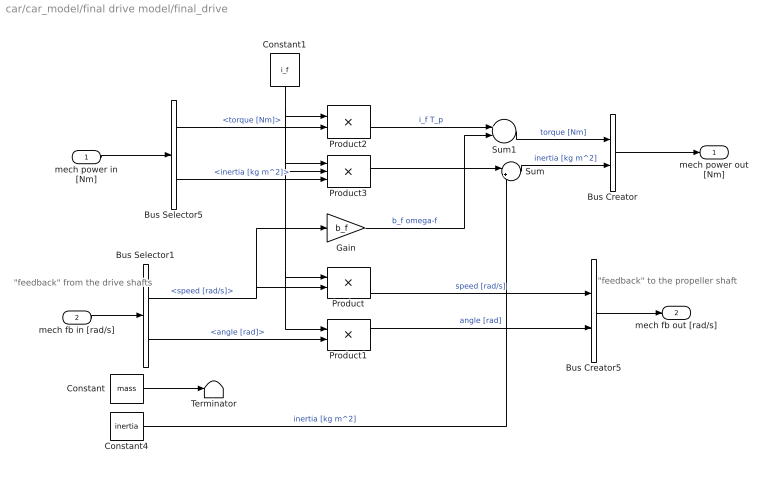
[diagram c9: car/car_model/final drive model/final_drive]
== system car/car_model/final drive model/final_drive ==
  note: "feedback" to the propeller shaft
  note: "feedback" from the drive shafts
  mech power in [Nm] : Inport  OutDataType=sfix(16)  OutScaling=2^0
  mech fb in [rad/s] : Inport  Port=2  OutDataType=sfix(16)  OutScaling=2^0
  Bus Creator : BusCreator  Inputs=2
  Bus Creator5 : BusCreator  Inputs=2
  Bus Selector1 : BusSelector  OutputSignals=speed [rad/s],angle [rad]
  Bus Selector5 : BusSelector  OutputSignals=torque [Nm],inertia [kg m^2]
  Constant : Constant  Value=mass  OutDataType=sfix(16)  OutScaling=2^0
  Constant1 : Constant  Orientation=down  Value=i_f  OutDataType=sfix(16)  OutScaling=2^0
  Constant4 : Constant  Value=inertia  OutDataType=sfix(16)  OutScaling=2^0
  Gain : Gain  Gain=b_f  ParameterDataType=sfix(16)  ParameterScaling=2^0  OutDataType=sfix(16)  OutScaling=2^0
  Product : Product  Inputs=**  OutDataType=sfix(16)  OutScaling=2^0
  Product1 : Product  Inputs=**  OutDataType=sfix(16)  OutScaling=2^0
  Product2 : Product  OutDataType=sfix(16)  OutScaling=2^0
  Product3 : Product  Inputs=3  OutDataType=sfix(16)  OutScaling=2^0
  Sum : Sum  Inputs=|++  OutDataType=sfix(16)  OutScaling=2^0
  Sum1 : Sum  Inputs=+-  OutDataType=sfix(16)  OutScaling=2^0
  Terminator : Terminator
  mech power out [Nm] : Outport  OutDataType=sfix(16)  OutScaling=2^0
  mech fb out [rad/s] : Outport  Port=2  OutDataType=sfix(16)  OutScaling=2^0
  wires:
  Gain/1 -> Sum1/2  "b_f omega-f"
  Sum1/1 -> Bus Creator/1  "torque [Nm]"
  Product2/1 -> Sum1/1  "i_f T_p"
  Sum/1 -> Bus Creator/2  "inertia [kg m^2]"
  Product3/1 -> Sum/1
  Constant4/1 -> Sum/2  "inertia [kg m^2]"
  Constant1/1 -> Product3/2, Product3/1, Product2/1, Product1/1, Product/1
  mech fb in [rad/s]/1 -> Bus Selector1/1
  Bus Creator/1 -> mech power out [Nm]/1
  Bus Selector1/2 -> Product1/2  "<angle [rad]>"
  Constant/1 -> Terminator/1
  Bus Selector1/1 -> Gain/1, Product/2  "<speed [rad/s]>"
  mech power in [Nm]/1 -> Bus Selector5/1
  Bus Selector5/1 -> Product2/2  "<torque [Nm]>"
  Bus Selector5/2 -> Product3/3  "<inertia [kg m^2]>"
  Product/1 -> Bus Creator5/1  "speed [rad/s]"
  Product1/1 -> Bus Creator5/2  "angle [rad]"
  Bus Creator5/1 -> mech fb out [rad/s]/1

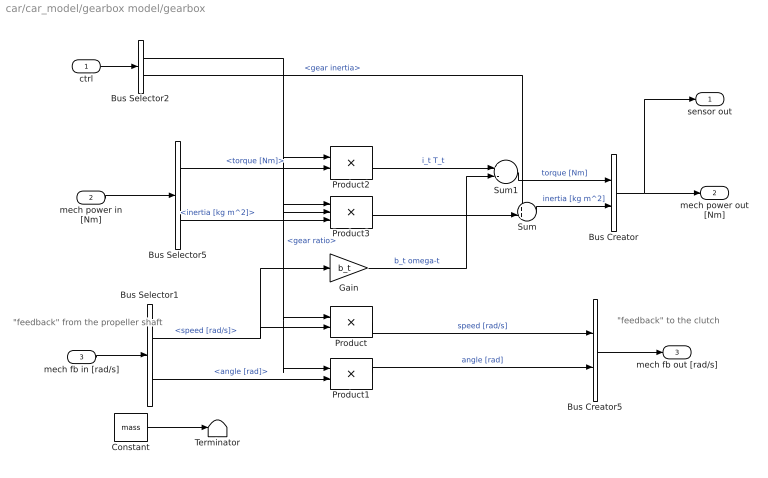
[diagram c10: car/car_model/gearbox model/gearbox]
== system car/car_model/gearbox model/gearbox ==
  note: "feedback" from the propeller shaft
  note: "feedback" to the clutch
  ctrl : Inport  OutDataType=sfix(16)  OutScaling=2^0
  mech power in [Nm] : Inport  Port=2  OutDataType=sfix(16)  OutScaling=2^0
  mech fb in [rad/s] : Inport  Port=3  OutDataType=sfix(16)  OutScaling=2^0
  Bus Creator : BusCreator  Inputs=2
  Bus Creator5 : BusCreator  Inputs=2
  Bus Selector1 : BusSelector  OutputSignals=speed [rad/s],angle [rad]
  Bus Selector2 : BusSelector  OutputSignals=gear ratio,gear inertia
  Bus Selector5 : BusSelector  OutputSignals=torque [Nm],inertia [kg m^2]
  Constant : Constant  Value=mass  OutDataType=sfix(16)  OutScaling=2^0
  Gain : Gain  Gain=b_t  ParameterDataType=sfix(16)  ParameterScaling=2^0  OutDataType=sfix(16)  OutScaling=2^0
  Product : Product  Inputs=**  OutDataType=sfix(16)  OutScaling=2^0
  Product1 : Product  Inputs=**  OutDataType=sfix(16)  OutScaling=2^0
  Product2 : Product  OutDataType=sfix(16)  OutScaling=2^0
  Product3 : Product  Inputs=3  OutDataType=sfix(16)  OutScaling=2^0
  Sum : Sum  Inputs=++|  OutDataType=sfix(16)  OutScaling=2^0
  Sum1 : Sum  Inputs=+-  OutDataType=sfix(16)  OutScaling=2^0
  Terminator : Terminator
  sensor out : Outport  OutDataType=sfix(16)  OutScaling=2^0
  mech power out [Nm] : Outport  Port=2  OutDataType=sfix(16)  OutScaling=2^0
  mech fb out [rad/s] : Outport  Port=3  OutDataType=sfix(16)  OutScaling=2^0
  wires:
  Bus Creator5/1 -> mech fb out [rad/s]/1
  Product1/1 -> Bus Creator5/2  "angle [rad]"
  Product/1 -> Bus Creator5/1  "speed [rad/s]"
  Bus Selector5/2 -> Product3/3  "<inertia [kg m^2]>"
  Bus Selector5/1 -> Product2/2  "<torque [Nm]>"
  mech power in [Nm]/1 -> Bus Selector5/1
  Bus Selector1/1 -> Product/2, Gain/1  "<speed [rad/s]>"
  Constant/1 -> Terminator/1
  Bus Selector1/2 -> Product1/2  "<angle [rad]>"
  Bus Creator/1 -> mech power out [Nm]/1, sensor out/1
  mech fb in [rad/s]/1 -> Bus Selector1/1
  ctrl/1 -> Bus Selector2/1
  Bus Selector2/1 -> Product2/1, Product3/1, Product3/2, Product/1, Product1/1  "<gear ratio>"
  Product2/1 -> Sum1/1  "i_t T_t"
  Sum1/1 -> Bus Creator/1  "torque [Nm]"
  Gain/1 -> Sum1/2  "b_t omega-t"
  Bus Selector2/2 -> Sum/1  "<gear inertia>"
  Sum/1 -> Bus Creator/2  "inertia [kg m^2]"
  Product3/1 -> Sum/2

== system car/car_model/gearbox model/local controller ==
  cmd in : Inport  OutDataType=sfix(16)  OutScaling=2^0
  sensor in : Inport  Port=2  OutDataType=sfix(16)  OutScaling=2^0
  Bus Creator : BusCreator  Inputs=2
  Bus Selector : BusSelector  OutputSignals=gear number
  gear number to inertia table : Lookup  InputValues=gearNumber  Table=gearInertia  LookUpMeth=Interpolation-Use End Values  OutDataType=sfix(16)  OutScaling=2^0
  gear number to ratio table : Lookup  InputValues=gearNumber  Table=gearRatio  LookUpMeth=Interpolation-Use End Values  OutDataType=sfix(16)  OutScaling=2^0
  sensor out : Outport  OutDataType=sfix(16)  OutScaling=2^0
  ctrl : Outport  Port=2  OutDataType=sfix(16)  OutScaling=2^0
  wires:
  sensor in/1 -> sensor out/1
  cmd in/1 -> Bus Selector/1
  Bus Selector/1 -> gear number to ratio table/1, gear number to inertia table/1  "<gear number>"
  Bus Creator/1 -> ctrl/1
  gear number to ratio table/1 -> Bus Creator/1  "gear ratio"
  gear number to inertia table/1 -> Bus Creator/2  "gear inertia"

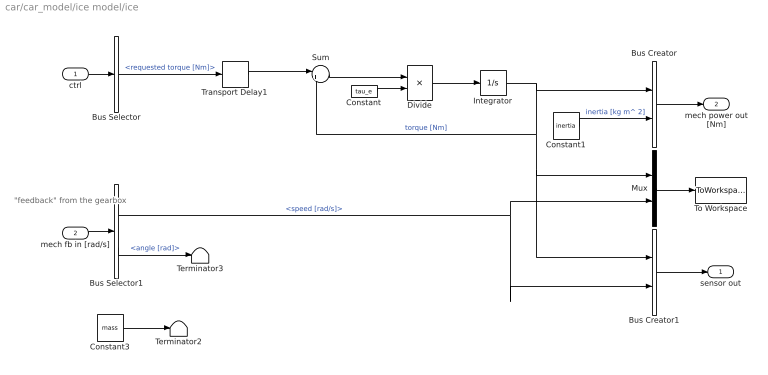
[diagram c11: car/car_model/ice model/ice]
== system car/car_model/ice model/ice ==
  note: "feedback" from the gearbox
  ctrl : Inport  OutDataType=sfix(16)  OutScaling=2^0
  mech fb in [rad/s] : Inport  Port=2  OutDataType=sfix(16)  OutScaling=2^0
  Bus Creator : BusCreator  Inputs=2
  Bus Creator1 : BusCreator  Inputs=2
  Bus Selector : BusSelector  OutputSignals=requested torque [Nm]
  Bus Selector1 : BusSelector  OutputSignals=speed [rad/s],angle [rad]
  Constant : Constant  Value=tau_e  OutDataType=sfix(16)  OutScaling=2^0
  Constant1 : Constant  Value=inertia  OutDataType=sfix(16)  OutScaling=2^0
  Constant3 : Constant  Value=mass  OutDataType=sfix(16)  OutScaling=2^0
  Divide : Product  Inputs=*/  OutDataType=sfix(16)  OutScaling=2^-10
  Integrator : Integrator  InitialCondition=init_T
  Mux : Mux  Inputs=2
  Sum : Sum  Inputs=|+-  OutDataType=sfix(16)  OutScaling=2^0
  Terminator2 : Terminator
  Terminator3 : Terminator
  To Workspace : ToWorkspace  VariableName=iceout  SampleTime=-1  SaveFormat=Array
  Transport Delay1 : TransportDelay  DelayTime=tau_d
  sensor out : Outport  OutDataType=sfix(16)  OutScaling=2^0
  mech power out [Nm] : Outport  Port=2  OutDataType=sfix(16)  OutScaling=2^0
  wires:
  Constant3/1 -> Terminator2/1
  Bus Creator1/1 -> sensor out/1
  Mux/1 -> To Workspace/1
  Bus Selector1/2 -> Terminator3/1  "<angle [rad]>"
  Bus Creator/1 -> mech power out [Nm]/1
  mech fb in [rad/s]/1 -> Bus Selector1/1
  ctrl/1 -> Bus Selector/1
  Constant/1 -> Divide/2
  Divide/1 -> Integrator/1
  Sum/1 -> Divide/1
  Integrator/1 -> Bus Creator/1, Sum/2, Mux/1, Bus Creator1/1  "torque [Nm]"
  Constant1/1 -> Bus Creator/2  "inertia [kg m^ 2]"
  Bus Selector1/1 -> Mux/2, Bus Creator1/2  "<speed [rad/s]>"
  Bus Selector/1 -> Transport Delay1/1  "<requested torque [Nm]>"
  Transport Delay1/1 -> Sum/1

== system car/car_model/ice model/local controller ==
  cmd in : Inport  OutDataType=sfix(16)  OutScaling=2^0
  sensor in : Inport  Port=2  OutDataType=sfix(16)  OutScaling=2^0
  Bus Creator : BusCreator  Inputs=1
  Bus Selector : BusSelector  OutputSignals=torque level
  Bus Selector1 : BusSelector  OutputSignals=speed [rad/s]
  Compare To Constant : simulink/Logic and Bit Operations/Compare To Constant  SystemSampleTime=-1  relop=<=  const=N_max  LogicOutDataTypeMode=uint8  ZeroCross=off
  Product : Product  OutDataType=sfix(16)  OutScaling=2^0
  Saturation : Saturate  UpperLimit=T_max  LowerLimit=-T_max
  gain : Gain  ParameterDataType=sfix(16)  ParameterScaling=2^0  OutDataType=sfix(16)  OutScaling=2^0
  sensor out : Outport  OutDataType=sfix(16)  OutScaling=2^0
  ctrl : Outport  Port=2  OutDataType=sfix(16)  OutScaling=2^0
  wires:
  cmd in/1 -> Bus Selector/1
  Bus Selector/1 -> Saturation/1  "<torque level>"
  Saturation/1 -> gain/1
  Bus Creator/1 -> ctrl/1
  sensor in/1 -> Bus Selector1/1, sensor out/1
  Product/1 -> Bus Creator/1  "requested torque [Nm]"
  gain/1 -> Product/1
  Bus Selector1/1 -> Compare To Constant/1  "<speed [rad/s]>"
  Compare To Constant/1 -> Product/2

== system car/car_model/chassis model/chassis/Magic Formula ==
  note: Note: The SAE definition of the slip ratio kappa is used.
  forward velocity [m/s] : Inport  OutDataType=sfix(16)  OutScaling=2^0
  wheel speed [rad/s] : Inport  Port=2  OutDataType=sfix(16)  OutScaling=2^0
  Constant : Constant  Orientation=down  OutDataType=sfix(16)  OutScaling=2^0
  Divide : Product  Inputs=*/  OutDataType=sfix(16)  OutScaling=2^-10
  Gain : Gain  Gain=r_w  ParameterDataType=sfix(16)  ParameterScaling=2^0  OutDataType=sfix(16)  OutScaling=2^0
  Magic Formula : Fcn  Expr=Dx*sin(Cx*atan(Bx*u-Ex*(Bx*u-atan(Bx*u))))
  Sum3 : Sum  Inputs=-+|  OutDataType=sfix(16)  OutScaling=2^0
  F_w [N] : Outport  OutDataType=sfix(16)  OutScaling=2^0
  slip ratio : Outport  Port=2  OutDataType=sfix(16)  OutScaling=2^0
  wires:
  Gain/1 -> Divide/1
  Sum3/1 -> Magic Formula/1, slip ratio/1  "kappa"
  Constant/1 -> Sum3/1
  Divide/1 -> Sum3/2
  wheel speed [rad/s]/1 -> Gain/1
  Magic Formula/1 -> F_w [N]/1
  forward velocity [m/s]/1 -> Divide/2
